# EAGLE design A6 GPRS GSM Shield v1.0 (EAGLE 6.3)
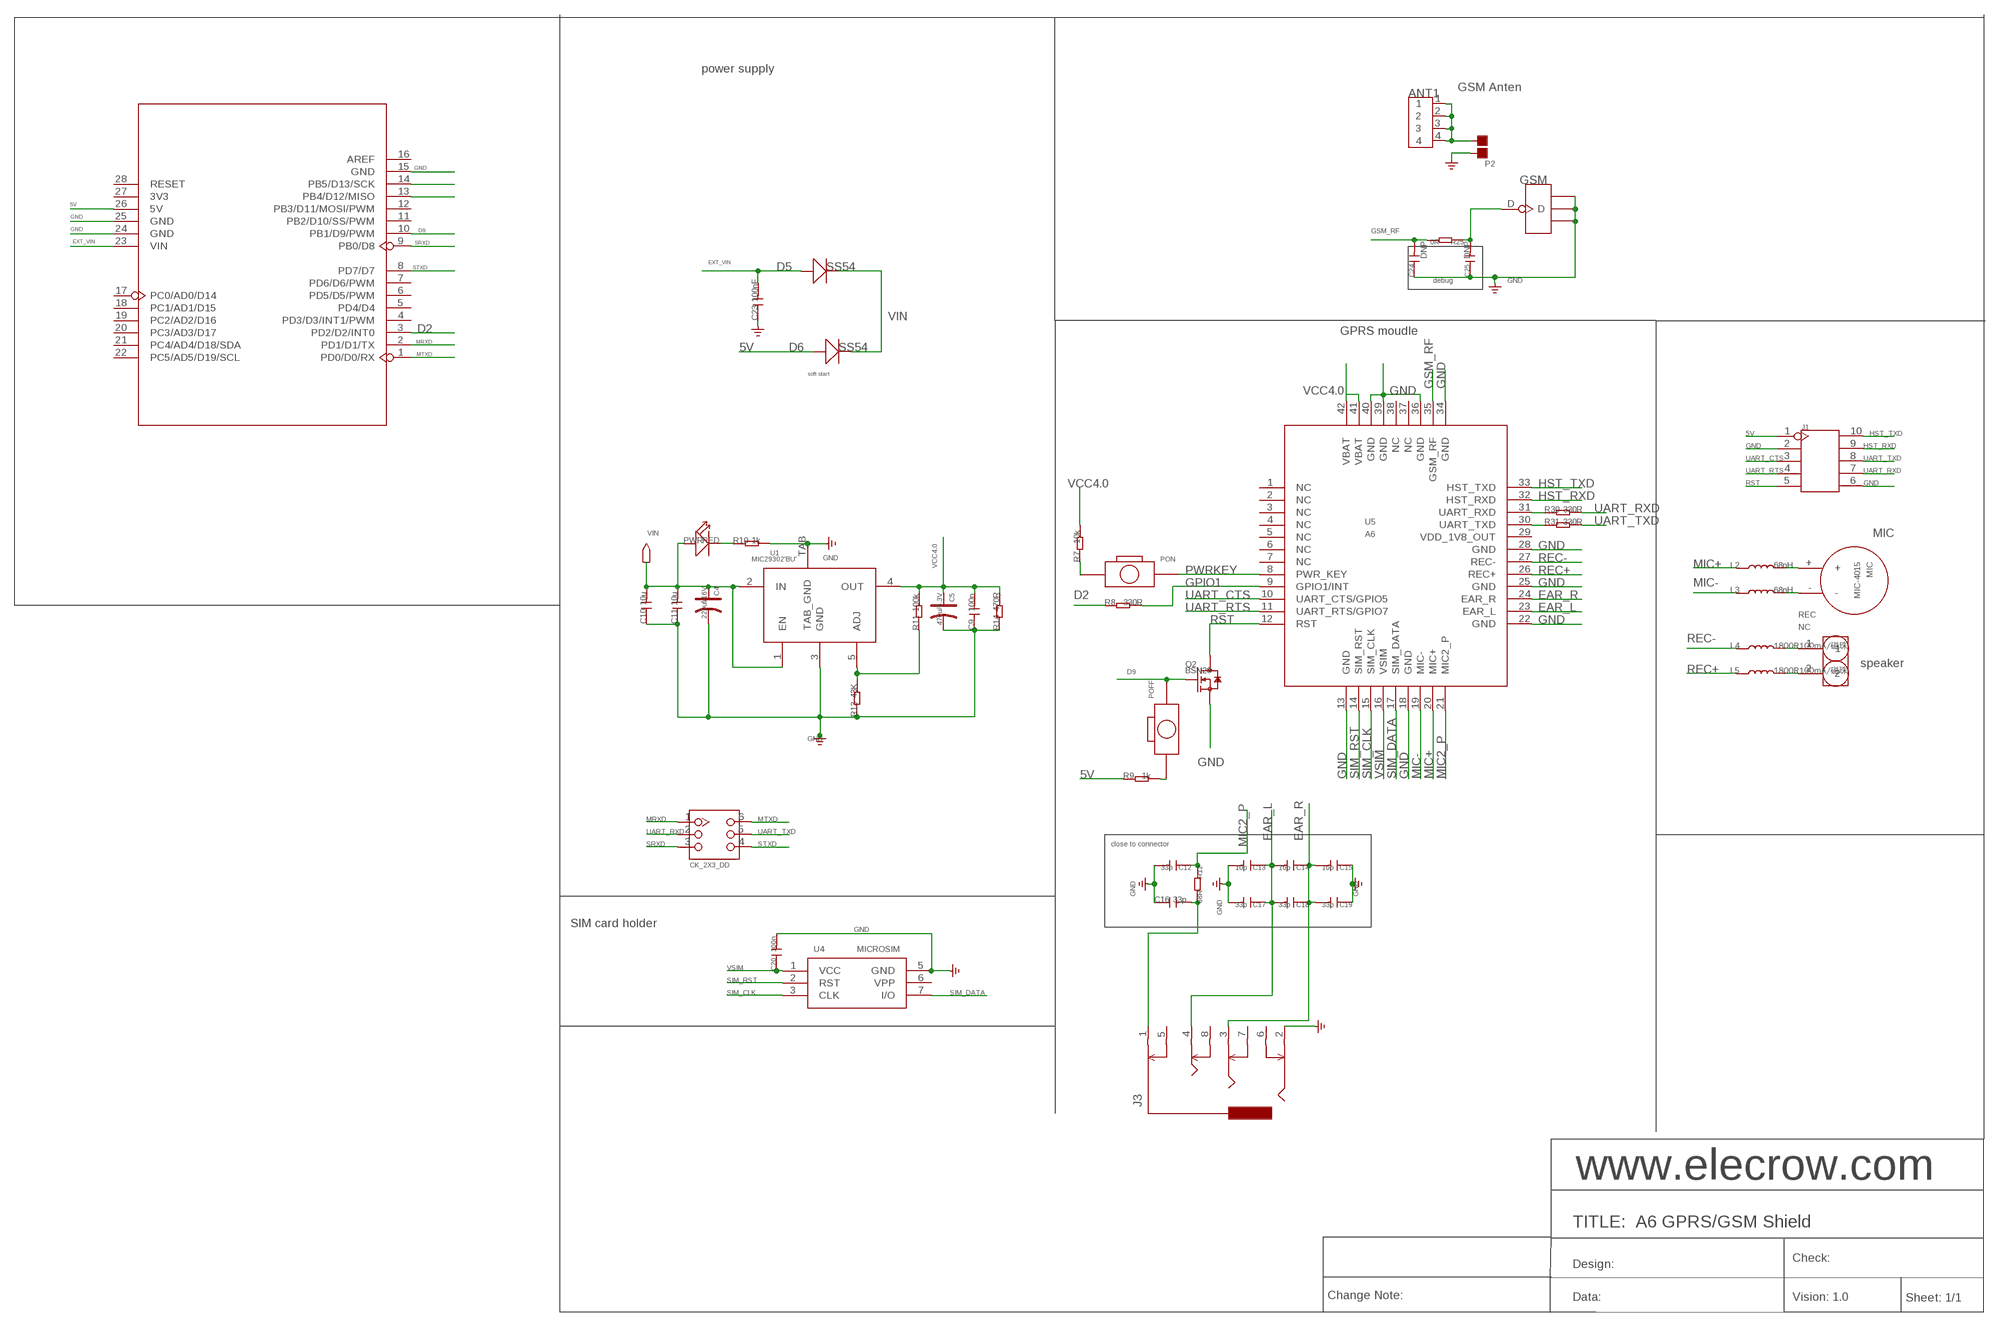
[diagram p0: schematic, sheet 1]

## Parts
ANT1  ANTENNA-SMA-IPX  [SMA-TO-IPX]
C4  220uf/16V  006-CAP_AVX_D  [AVX_D]
C5  470u/6.3V  006-CAP_AVX_D  [AVX_D]
C9  100n  C-0603  [C0603]
C10  10u  C-0603  [C0603]
C11  10u  C-0603  [C0603]
C12  33p  C-0603  [C0603]
C13  10p  C-0402  [C0402]
C14  10p  C-0402  [C0402]
C15  10p  C-0402  [C0402]
C16  33p  C-0603  [C0603]
C17  33p  C-0402  [C0402]
C18  33p  C-0402  [C0402]
C19  33p  C-0402  [C0402]
C20  100n  C-0603  [C0603]
C23  100nF  C-0603  [C0603]
C24  DNP  C-0402  [C0402]
C25  DNP  C-0402  [C0402]
D5  SS54  D'MBRS240LT3'  [SMB]
D6  SS54  D'MBRS240LT3'  [SMB]
GSM  ANTENNA-U-FL  [4P-U-FL]
J1  HEADER-2X5P-2.54  [2X5P-2.54]
J3  AUDIO-8P'PJ-3536-L6S'  [8P-3.5-SMD]
J7  CK_2X3_DD  [CK_2X3]
L2  68nH  L'0402'  [L0402]
L3  68nH  L'0402'  [L0402]
L4  1800R100mA/磁珠  L'0402'  [L0402]
L5  1800R100mA/磁珠  L'0402'  [L0402]
MIC  MIC-4015  [MIC-4015]
P2  PAD-JUMPER-2P  [2P-SMD-1.78X1.27]
POFF  BOTTON_1_DP  [BTN_5.0_RST]
PON  BOTTON_1_DP  [BTN_5.0_RST]
PWR  RED  007-LED0603  [D0603]
Q2  BSN20  MOSFET-N'SOT23'  [SOT23@1]
R7  10k  R-0603  [R0603]
R8  330R  R-0603  [R0603]
R9  1k  R-0603  [R0603]
R10  1k  R-0603  [R0603]
R11  100k  R-0603  [R0603]
R12  68R  R-0603  [R0603]
R13  43K  R-0603  [R0603]
R14  470R  R-0603  [R0603]
R25  0R  R-0402  [R0402]
R30  330R  R-0603  [R0603]
R31  330R  R-0603  [R0603]
REC  NC  HEADER-2P-65/35MIL  [2P-2.54-65/35MIL]
U1  MIC29302'BU'  [TO-263]
U3  UNO-SHILED  [SHILED]
U4  MICROSIM  [MICROSIM]
U5  A6  [A6]

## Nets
5V: D6.+ J1.1 R9.1 U3.26(5V)
D2: R8.1 U3.3(PD2/D2/INT0)
D9: POFF.P$2 Q2.1(G) U3.10(PB1/D9/PWM)
EAR_L: C13.1 C14.2 C17.1 C18.2 J3.4 U5.23(EAR_L)
EAR_R: C14.1 C15.2 C18.1 C19.2 J3.3 U5.24(EAR_R)
EXT_VIN: C23.2 D5.+ U3.23(VIN)
GND: C4.- C5.- C9.1 C10.1 C11.1 C12.2 C13.2 C15.1 C16.1 C17.2 C19.1 C20.2 C23.1 C24.1 C25.1 GSM.GND1 GSM.GND2 GSM.GND3 J1.2 J1.6 J3.2 P2.2 Q2.2(S) R10.2 R13.1 R14.1 U1.3(GND) U1.TAB(TAB_GND) U3.15(GND) U3.24(GND) U3.25(GND) U4.5(GND) U5.13(GND) U5.18(GND) U5.22(GND) U5.25(GND) U5.28(GND) U5.34(GND) U5.36(GND) U5.39(GND) U5.40(GND)
GPIO1: R8.2 U5.9(GPIO1/INT)
GSM_RF: C24.2 R25.2 U5.35(GSM_RF)
HST_RXD: J1.9 U5.32(HST_RXD)
HST_TXD: J1.10 U5.33(HST_TXD)
MIC2_P: C12.1 R12.1 U5.21(MIC2_P)
MIC+: L2.1 U5.20(MIC+)
MIC-: L3.1 U5.19(MIC-)
MRXD: J7.1 U3.2(PD1/D1/TX)
MTXD: J7.6 U3.1(PD0/D0/RX)
N$1: POFF.P$1 R9.2
N$2: R30.1 U5.31(UART_RXD)
N$4: R31.1 U5.30(UART_TXD)
N$5: R11.1 R13.2 U1.5(ADJ)
N$6: L3.2 MIC.-
N$7: PON.P$1 R7.1
N$8: L2.2 MIC.+
N$9: L4.2 REC.1
N$12: ANT1.1 ANT1.2 ANT1.3 ANT1.4 P2.1
N$17: L5.2 REC.2
N$19: PWR.- R10.1
N$23: U3.14(PB5/D13/SCK)
N$25: C25.2 GSM.D R25.1
N$27: U3.13(PB4/D12/MISO)
N$30: C16.2 J3.1 R12.2
PWRKEY: PON.P$2 U5.8(PWR_KEY)
REC+: L5.1 U5.26(REC+)
REC-: L4.1 U5.27(REC-)
RST: J1.5 Q2.3(D) U5.12(RST)
SIM_CLK: U4.3(CLK) U5.15(SIM_CLK)
SIM_DATA: U4.7(I/O) U5.17(SIM_DATA)
SIM_RST: U4.2(RST) U5.14(SIM_RST)
SRXD: J7.3 U3.9(PB0/D8)
STXD: J7.4 U3.8(PD7/D7)
UART_CTS: J1.3 U5.10(UART_CTS/GPIO5)
UART_RTS: J1.4 U5.11(UART_RTS/GPIO7)
UART_RXD: J1.7 J7.2 R30.2
UART_TXD: J1.8 J7.5 R31.2
VCC4.0: C5.+ C9.2 R7.2 R11.2 R14.2 U1.4(OUT) U5.41(VBAT) U5.42(VBAT)
VIN: C4.+ C10.2 C11.2 D5.- D6.- PWR.+ U1.1(EN) U1.2(IN)
VSIM: C20.1 U4.1(VCC) U5.16(VSIM)
Unconnected: J3.5 J3.6 J3.7 J3.8 U3.4(PD3/D3/INT1/PWM) U3.5(PD4/D4) U3.6(PD5/D5/PWM) U3.7(PD6/D6/PWM) U3.11(PB2/D10/SS/PWM) U3.12(PB3/D11/MOSI/PWM) U3.16(AREF) U3.17(PC0/AD0/D14) U3.18(PC1/AD1/D15) U3.19(PC2/AD2/D16) U3.20(PC3/AD3/D17) U3.21(PC4/AD4/D18/SDA) U3.22(PC5/AD5/D19/SCL) U3.27(3V3) U3.28(RESET) U4.6(VPP) U5.1(NC) U5.2(NC) U5.3(NC) U5.4(NC) U5.5(NC) U5.6(NC) U5.7(NC) U5.29(VDD_1V8_OUT) U5.37(NC) U5.38(NC)

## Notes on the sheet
- power supply
- GSM Anten
- debug
- GPRS moudle
- soft start
- MIC
- speaker
- close to connector
- SIM card holder
- www.elecrow.com
- TITLE:  A6 GPRS/GSM Shield
- Check:
- Design:
- Change Note: | Data: | Vision: 1.0 | Sheet: 1/1

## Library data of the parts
ANT1 = Connector:ANTENNA-SMA-IPX
C4 C5 = Discrete:006-CAP*: Electrolytic Capacitors,Tantalum Capacitors and Super Capacitors
C9-C20 C23-C25 = Discrete:C*: Ceramic Capacitors
D5 D6 = Discrete:D*
GSM = Connector:ANTENNA-U-FL
J1 = Connector:HEADER-2X5P
J3 = template:AUDIO-8P
J7 = CONNECTER:CK_2X3
L2-L5 = Discrete:L*
MIC = Discrete:MIC-4015
P2 = Discrete:PAD-JUMPER-2P; PARTNO: DNP
POFF PON = CPT_SMD:BOTTON_1
PWR = Discrete:007-LED*
Q2 = Discrete:MOSFET-N: IRLL014: http://www.vishay.com/docs/91319/sihll014.pdf
R7-R14 R25 R30 R31 = Discrete:R*
REC = Connector:HEADER-2P
U1 = ICs_v54:MIC29302
U3 = ljb:UNO-SHILED
U4 = Connector:MICROSIM
U5 = IC:A6

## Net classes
0 default: width 0.152 mm, drill 0.152 mm, clearance 0.152 mm
2 gnd: width 0.305 mm, drill 0.559 mm, clearance 0.254 mm

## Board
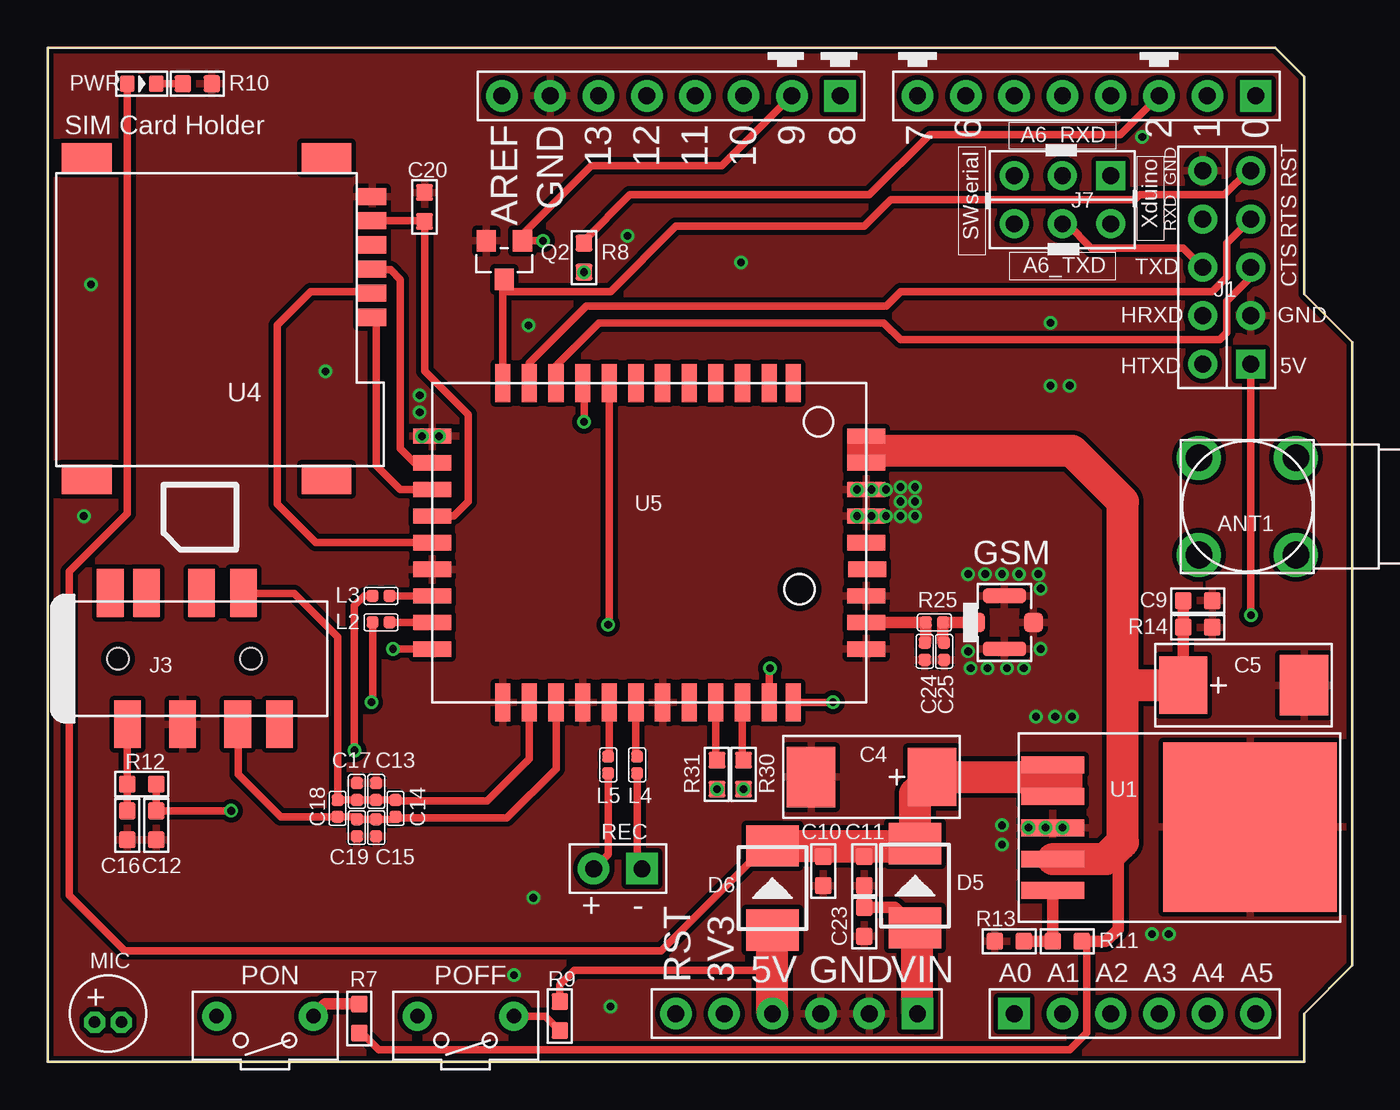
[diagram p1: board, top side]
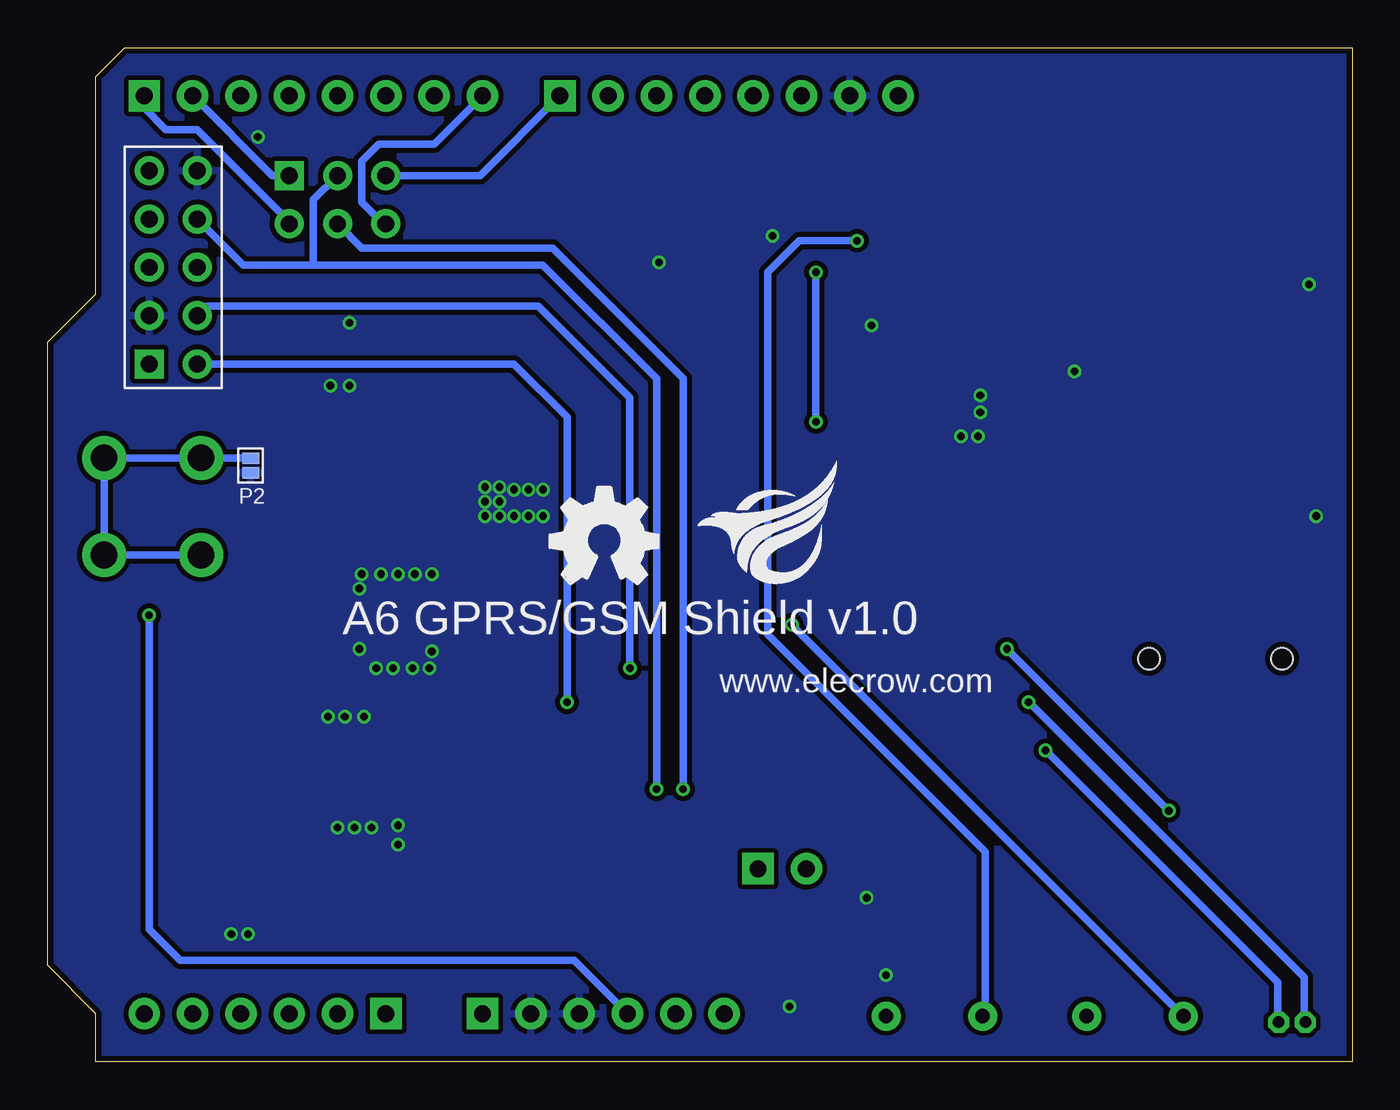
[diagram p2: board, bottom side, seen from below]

Size 68.58 x 53.34 mm. Coordinates in mm from the lower left corner, seen from the top.
Outline: 0,0 66.04,0 66.04,2.54 68.58,5.08 68.58,37.85 66.04,40.39 66.04,51.82 64.52,53.34 0,53.34 0,0
Copper layers (1*16): Top 0.035mm / dielectric 1.5mm / Bottom 0.035mm
Design rules "default *": minimum track width 6mil, minimum drill 12mil, track to track 10mil, track to pad 10mil, pad to pad 10mil, via to via 6mil, smd to smd 0mil, copper to edge 12mil, drill to drill 12mil, minimum pad ring 10mil, minimum via ring 6mil, stop-mask expansion 2mil, vias tented up to drill 100mil, thermal gap 10mil

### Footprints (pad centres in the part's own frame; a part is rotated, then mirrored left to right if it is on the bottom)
SMA-TO-IPX = drill 1.4 pad 2.3: 1 -2.55,2.55; 2 2.55,2.55; 3 2.55,-2.55; 4 -2.55,-2.55
AVX_D = smd 2.54 x 3.048: + -3.175,0 | smd 2.54 x 3.175: - 3.175,0
C0603 = smd 0.889 x 0.889: 1 -0.762,0; 2 0.762,0
C0402 = smd 0.635 x 0.635: 1 -0.445,0; 2 0.445,0
SMB = smd 2.159 x 2.743: + -2.21,0; - 2.21,0
4P-U-FL = smd 1.016 x 1.016: D -1.524,0; GND3 1.524,0 | smd 2.286 x 0.762: GND1 0,1.397; GND2 0,-1.397
2X5P-2.54-LEADED = drill 0.889 pad 1.524 square: 1 -1.27,5.08 | drill 0.889 pad 1.524: 2 -1.27,2.54; 3 -1.27,0; 4 -1.27,-2.54; 5 -1.27,-5.08; 6 1.27,-5.08; 7 1.27,-2.54; 8 1.27,0; 9 1.27,2.54; 10 1.27,5.08
8P-3.5-SMD = smd 1.4 x 2.5: 1 2.8,-3.45; 2 5.7,-3.45; 3 8.6,-3.45; 4 8.9,3.45; 5 1.9,3.45; 6 3.8,3.45; 7 6.7,3.45; 8 10.8,-3.45 | hole 1.149: 2.3,0; 9.3,0
CK_2X3 = drill 0.889 pad 1.524 square: 1 -1.27,2.54 | drill 0.889 pad 1.524: 2 -1.27,0; 3 -1.27,-2.54; 4 1.27,-2.54; 5 1.27,0; 6 1.27,2.54
L0402 = smd 0.635 x 0.635: 1 -0.445,0; 2 0.445,0
MIC-4015 = drill 0.6 octagon: + 0.7,0.45; - -0.7,0.45
2P-SMD-1.78X1.27 = smd 0.889 x 0.61: 1 0,0.381; 2 0,-0.381
BTN_5.0_RST = drill 0.762 pad 1.524: P$1 0,2.54; P$2 0,-2.54
D0603 = smd 0.762 x 0.889: + -0.762,0; - 0.762,0
SOT23@1 = smd 1.016 x 1.143: 1 -0.95,-1.016; 2 0.95,-1.016; 3 0,1.016
R0603 = smd 0.889 x 0.889: 1 -0.762,0; 2 0.762,0
R0402 = smd 0.635 x 0.635: 1 -0.445,0; 2 0.445,0
2P-2.54-65/35MIL = drill 0.889 pad 1.651 square: 1 0,1.27 | drill 0.889 pad 1.651: 2 0,-1.27
TO-263 = smd 3.302 x 0.889: 1 3.302,-3.302; 2 3.302,-1.651; 3 3.302,0; 4 3.302,1.651; 5 3.302,3.302 | smd 9.12 x 8.89: TAB -7.071,-0.03
SHILED = drill 0.889 pad 1.651 square: 1 63.5,50.8; 9 41.656,50.8; 17 50.8,2.54; 23 45.72,2.54 | drill 0.889 pad 1.651: 2 60.96,50.8; 3 58.42,50.8; 4 55.88,50.8; 5 53.34,50.8; 6 50.8,50.8; 7 48.26,50.8; 8 45.72,50.8; 10 39.116,50.8; 11 36.576,50.8; 12 34.036,50.8; 13 31.496,50.8; 14 28.956,50.8; 15 26.416,50.8; 16 23.876,50.8; 18 53.34,2.54; 19 55.88,2.54; 20 58.42,2.54; 21 60.96,2.54; 22 63.5,2.54; 24 43.18,2.54; 25 40.64,2.54; 26 38.1,2.54; 27 35.56,2.54; 28 33.02,2.54
MICROSIM = smd 1.5 x 0.9: 1 -0.8,2.5; 2 -0.8,5.04; 3 -0.8,7.58; 5 -0.8,1.23; 6 -0.8,3.77; 7 -0.8,6.31 | smd 2.61 x 1.56: P$1 1.6,-0.8; P$2 14.2,-0.8; P$3 14.2,16.1; P$4 1.6,16.1
A6 = smd 0.8 x 2: 1 7.57,8.4; 2 6.3,8.4; 3 4.9,8.4; 4 3.5,8.4; 5 2.1,8.4; 6 0.7,8.4; 7 -0.7,8.4; 8 -2.1,8.4; 9 -3.5,8.4; 10 -4.9,8.4; 11 -6.3,8.4; 12 -7.7,8.4; 22 -7.7,-8.4; 23 -6.3,-8.4; 24 -4.9,-8.4; 25 -3.5,-8.4; 26 -2.1,-8.4; 27 -0.7,-8.4; 28 0.7,-8.4; 29 2.1,-8.4; 30 3.5,-8.4; 31 4.9,-8.4; 32 6.3,-8.4; 33 7.57,-8.4 | smd 2 x 0.8: 13 -11.4,5.6; 14 -11.4,4.2; 15 -11.4,2.8; 16 -11.4,1.4; 17 -11.4,0; 18 -11.4,-1.4; 19 -11.4,-2.8; 20 -11.4,-4.2; 21 -11.4,-5.6; 34 11.4,-5.6; 35 11.4,-4.2; 36 11.4,-2.8; 37 11.46,-1.4; 38 11.4,0; 39 11.4,1.4; 40 11.4,2.8; 41 11.4,4.2; 42 11.4,5.6

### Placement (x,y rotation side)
ANT1  63.06,29.21 90 top
C4  43.31,14.99 180 top
C5  62.87,19.81 0 top
C9  60.45,24.26 180 top
C10  40.77,10.03 90 top
C11  42.93,10.03 90 top
C12  5.71,12.45 270 top
C13  17.27,14.22 90 top
C14  18.29,13.34 90 top
C15  17.27,12.32 90 top
C16  4.19,12.45 90 top
C17  16.26,14.22 90 top
C18  15.24,13.34 90 top
C19  16.26,12.32 90 top
C20  19.81,44.96 90 top
C23  42.93,7.37 90 top
C24  46.1,21.59 90 top
C25  47.12,21.59 90 top
D5  45.59,9.27 90 top
D6  38.1,9.14 90 top
GSM  50.29,23.11 0 top
J1  [2X5P-2.54-LEADED]  61.98,41.78 180 top
J3  1.4,21.21 0 top
J7  53.34,45.34 270 top
L2  17.53,23.11 180 top
L3  17.53,24.51 180 top
L4  30.99,15.62 270 top
L5  29.46,15.62 270 top
LOGO2  LOGO-OSHW-FILLX0200-NT  [OSHW_FILLX200_NOTEXT]  42.16,25.15 0 bottom
MIC  3.17,2.54 180 top
P2  57.91,31.37 0 bottom
POFF  21.97,2.41 270 top
PON  11.43,2.41 270 top
PWR  4.95,51.44 0 top
Q2  24,42.16 180 top
R7  16.38,2.29 270 top
R8  28.19,42.29 270 top
R9  26.92,2.41 270 top
R10  7.87,51.44 0 top
R11  53.59,6.35 0 top
R12  4.95,14.61 180 top
R13  50.55,6.35 0 top
R14  60.45,22.86 180 top
R25  46.61,23.11 180 top
R30  36.58,15.11 270 top
R31  35.18,15.11 270 top
REC  29.97,10.16 270 top
U1  56.13,12.32 180 top
U3  0,0 0 top
U4  16.26,46.74 180 top
U5  31.62,27.3 0 top
U$4  [ELECROW_NRW_6]  34.42,25.15 0 bottom

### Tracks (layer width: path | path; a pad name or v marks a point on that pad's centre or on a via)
5V  (via drill 0.41)
  Top 0.406: R9.1 26.92,4.06 27.69,4.83 37.97,4.83 38.1,4.7 | J1.1 v63.25,23.5
  Top 1.676: U3.26 38.1,4.7 D6.+
  Bottom 0.406: v63.25,23.5 63.25,6.99 61.59,5.33 40.89,5.33 U3.26
D2
  Top 0.406: R8.1 28.19,43.18 30.61,45.59 43.18,45.59 46.35,48.77 56.39,48.77 U3.3
D9  (via drill 0.41)
  Top 0.406: U3.10 35.43,47.12 28.57,47.12 24.95,43.49 Q2.1 v26.04,43.18
  Bottom 0.406: v26.04,43.18 29.08,43.18 30.73,41.53 30.73,22.48 19.3,11.05 19.3,2.54 POFF.P$2
EAR_L
  Top 0.406: U5.23 25.32,15.93 23.11,13.72 18.35,13.72 C14.2 C13.1 C17.1 C18.2 15.24,22.35 12.95,24.64 10.32,24.64 J3.4
EAR_R
  Top 0.406: J3.3 10.03,17.72 10.03,15.11 12.26,12.89 C18.1 16.13,12.89 C19.2 C15.2 18.16,12.76 C14.1 18.35,12.83 24.13,12.83 26.72,15.42 U5.24
EXT_VIN
  Top 0.61: C23.2 44.53,8.13 D5.+
  Top 1.676: U3.23 45.72,6.93 D5.+
GND  (via drill 0.41)
  other vias: 51.31,20.7 50.42,20.7 49.4,20.7 48.51,20.7 48.39,21.59 52.2,21.72 52.2,24.89 52.07,25.65 51.05,25.65 50.16,25.65 49.28,25.65 48.39,25.65 44.83,30.23 44.83,29.46 44.83,28.7 42.55,30.1 43.31,30.1 44.07,30.1 42.55,28.7 43.31,28.7 44.07,28.7 45.59,30.23 45.59,29.46 45.59,28.7 52.7,35.56 52.7,38.86 53.72,35.56 36.45,42.04 30.48,43.43 25.27,38.73 14.61,36.32 19.56,35.05 19.56,34.16 19.68,32.89 20.57,32.89 25.53,8.64 57.53,48.64 29.59,2.92 24.51,4.57 2.29,40.89 1.91,28.7 51.56,12.32 52.45,12.32 53.34,12.32 50.16,12.45 50.16,11.43 51.94,18.16 52.96,18.16 53.85,18.16 58.93,6.73 58.04,6.73
  pour Bottom (isolate 0.254): -1.27,-1.27 71.12,-1.27 71.12,54.61 -1.27,54.61
  pour Top (isolate 0.254): -1.27,-1.27 71.12,-1.27 71.12,54.61 -1.27,54.61
GPIO1  (via drill 0.41)
  Top 0.406: U5.9 28.19,35.78 v28.19,33.66
  Bottom 0.406: v28.19,33.66 R8.2
  other vias: 28.19,41.53
GSM_RF
  Top 0.61: U5.35 R25.2 46.16,22.1 C24.2
HST_RXD  (via drill 0.41)
  Top 0.406: U5.32 37.92,20.65 v37.97,20.7
  Bottom 0.406: v37.97,20.7 37.97,34.92 42.8,39.75 60.2,39.75 J1.9
HST_TXD  (via drill 0.41)
  Top 0.406: U5.33 41.26,18.91 v41.27,18.92
  Bottom 0.406: v41.27,18.92 41.27,33.91 44.07,36.7 J1.10
MIC2_P  (via drill 0.41)
  Top 0.406: R12.1 C12.1 v9.65,13.21 | U5.21 18.17,21.7 v18.16,21.72
  Bottom 0.406: v18.16,21.72 v9.65,13.21
MIC+
  Top 0.406: U5.20 L2.1
MIC-
  Top 0.406: U5.19 L3.1
MRXD
  Bottom 0.406: J7.1 56.77,46.61 U3.2
MTXD
  Bottom 0.406: J7.6 55.88,44.2 60.71,49.02 62.36,49.02 63.5,50.16 U3.1
N$1
  Top 0.406: POFF.P$1 26.16,2.41 R9.2
N$2
  Top 0.406: U5.31 36.52,15.93 R30.1
N$4
  Top 0.406: U5.30 35.12,15.93 R31.1
N$5
  Top 0.61: U1.5 R11.1 R13.2
N$6  (via drill 0.41)
  Top 0.406: L3.2 16.64,24.51 16.13,24 v16.13,16.38
  Bottom 0.406: v16.13,16.38 3.94,4.19 3.94,2.15 MIC.-
N$7
  Top 0.61: R7.1 14.61,3.05 PON.P$1
N$8  (via drill 0.41)
  Top 0.406: L2.2 17.08,18.99 v17.02,18.92
  Bottom 0.406: v17.02,18.92 2.54,4.45 2.54,2.15 MIC.+
N$9
  Top 0.406: L4.2 30.99,10.41 REC.1
N$12
  Bottom 0.406: ANT1.1 ANT1.4 ANT1.3 ANT1.2 57.92,31.76 P2.1
N$17
  Top 0.406: L5.2 29.46,10.92 REC.2
N$19
  Top 0.406: PWR.- R10.1
N$25
  Top 0.61: C25.2 47.05,22.1 R25.1 GSM.D
N$30
  Top 0.406: C16.2 R12.2 J3.1
PWRKEY  (via drill 0.41)
  Top 0.406: U5.8 29.52,23.05 v29.46,22.99
  Bottom 0.406: v29.46,22.99 PON.P$2
REC+
  Top 0.406: U5.26 29.52,16.12 L5.1
REC-
  Top 0.406: U5.27 30.92,16.13 L4.1
RST
  Top 0.406: U5.12 23.92,40.39 | 23.92,40.39 23.92,41.07 Q2.3 | J1.5 63.12,46.86 61.85,45.59 57.4,45.59 57.15,45.34 44.32,45.34 42.93,43.94 33.02,43.94 29.59,40.51 24.05,40.51 23.92,40.39
SIM_CLK
  Top 0.406: U5.15 18.54,30.11 17.27,31.37 17.27,38.94 U4.3
SIM_DATA
  Top 0.406: U5.17 14.1,27.3 12.06,29.34 12.06,38.73 13.84,40.51 16.97,40.51 U4.7
SIM_RST
  Top 0.406: U5.14 19.3,31.5 18.54,32.26 18.54,41.15 18.03,41.66 17.1,41.66 U4.2
SRXD
  Bottom 0.406: J7.3 45.85,46.61 U3.9
STXD
  Bottom 0.406: J7.4 50.93,44.07 52.07,45.21 52.07,47.37 51.18,48.26 48.26,48.26 U3.8
UART_CTS
  Top 0.406: U5.10 26.72,36.63 28.96,38.86 43.94,38.86 44.83,37.97 61.59,37.97 61.98,38.35 61.98,40.01 63.25,41.27 J1.3
UART_RTS
  Top 0.406: U5.11 25.32,36.75 28.32,39.75 44.07,39.75 44.83,40.51 61.21,40.51 61.98,41.27 61.98,43.05 J1.4
UART_RXD  (via drill 0.41)
  Bottom 0.406: R30.2 36.58,35.94 42.55,41.91 54.74,41.91 | 54.74,41.91 58.29,41.91 J1.7 | J7.2 54.61,45.34 54.61,42.04 54.74,41.91
  other vias: 36.58,14.35
UART_TXD  (via drill 0.41)
  Top 0.406: J7.5 53.59,44.07 54.86,42.8 59.69,42.8 J1.8
  Bottom 0.406: R31.2 35.18,35.94 42.04,42.8 52.07,42.8 J7.5
  other vias: 35.18,14.35
VCC4.0
  Top 0.406: R7.2 16.51,1.52 17.4,0.64 53.72,0.64 54.61,1.52 54.61,6.1 R11.2 | 43.03,32.89 U5.42 43.02,32.13 U5.41
  Top 0.61: R11.2 55.63,6.35 56.26,6.99 56.26,11.3 56.39,11.43 | C5.+ R14.2 C9.2
  Top 1.676: U1.4 55.63,10.67 56.39,11.43 56.52,11.56 56.52,19.56 | 56.52,19.56 56.52,29.46 53.85,32.13 43.02,32.13 | C5.+ 56.77,19.81 56.52,19.56
VIN
  Top 0.406: D6.- 37.77,11.35 32.26,5.84 4.06,5.84 1.14,8.76 1.14,25.78 4.19,28.83 PWR.+
  Top 0.61: U1.2 52.96,14.1 54.1,14.1 54.1,15.62 U1.1 53.21,15.62 53.85,14.99 53.85,14.73 53.59,14.48 53.21,14.48 52.83,14.86 | C10.2 C11.2 44.91,10.79 D5.-
  Top 1.676: 52.83,14.86 52.7,14.99 C4.+ 45.59,14.1 D5.- 45.47,11.35 D6.-
VSIM
  Top 0.406: U4.1 19.77,44.24 C20.1 19.81,36.32 22.1,34.04 22.1,29.46 21.34,28.7 U5.16
(copper drawn outside any net)
  shapes: Top area x1

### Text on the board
tPlace: 6 | 2 | 1 | 0 | SIM Card Holder | 13 | 12 | 11 | 10 | 9 | 8 | 7 | A6_RXD | SWserial | Xduino | GND | RST | RXD | RTS | A6_TXD | TXD | CTS | HRXD | GND | HTXD | 5V | + | -
bPlace: A6 GPRS/GSM Shield v1.0 | www.elecrow.com
tNames: AREF | GND | RST | 3V3 | 5V | GND | VIN | A0 | A1 | A2 | A3 | A4 | A5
